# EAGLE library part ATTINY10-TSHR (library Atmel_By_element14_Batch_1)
8-bit Microcontroller with In-System Programmable Flash
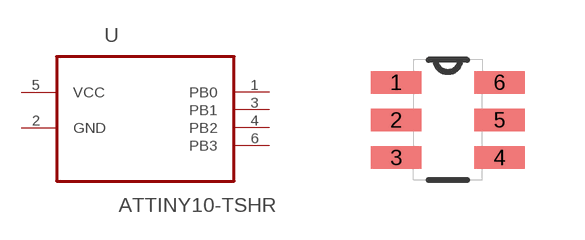
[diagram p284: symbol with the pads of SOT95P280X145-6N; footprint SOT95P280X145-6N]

Designator prefix U

## ATTINY10-TSHR (MPN: ATTINY10-TSHR; OC_FARNELL: 1748538; OC_NEWARK: 26R5645; PACKAGE: SOT-23-6; SUPPLIER: Atmel)  [SOT95P280X145-6N]
1  PB0
2  GND  pas
3  PB1
4  PB2
5  VCC  pwr
6  PB3

## Footprint SOT95P280X145-6N (pad centres in mm)
smd 1.27 x 0.559: 1 -1.295,0.94; 2 -1.295,0; 3 -1.295,-0.94; 4 1.295,-0.94; 5 1.295,0; 6 1.295,0.94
